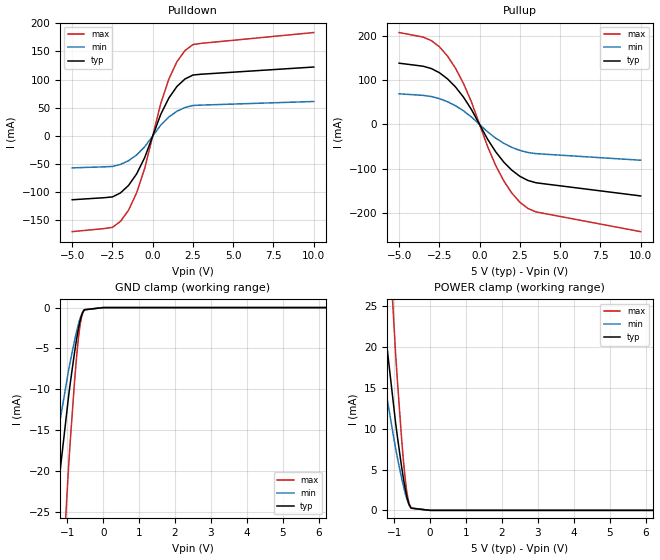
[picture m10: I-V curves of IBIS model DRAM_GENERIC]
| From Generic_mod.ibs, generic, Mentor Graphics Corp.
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[Model]   DRAM_GENERIC
Model_type   I/O
Polarity   Non-Inverting
Vinl  =   0.800V
Vinh  =   2.000V
Vmeas =   1.500V
Cref  =  50.000pF
Rref  =   1.000kOhm
Vref  =   0.000V
|   typ   min   max
C_comp   5.000pF   2.500pF   7.500pF
[Voltage Range]   5.000V   4.500V   5.500V
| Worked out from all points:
|   slope of the pulldown table from 0 to 0.75 V, typ, clamps not added: 14.2 ohm
|   slope of the pullup table from 0 to 0.75 V, typ, clamps not added: 15.8 ohm
|   GND clamp passes 1 mA (typ) near -0.61 V on its own axis
|   POWER clamp passes 1 mA (typ) near -0.61 V on its own axis
[Pulldown]
| Voltage   I(typ)   I(min)   I(max)
-5V       -113.2mA   -56.6mA    -169.8mA
-2.5V     -108.2mA   -54.08mA   -162.2mA
-2V       -101mA     -50.51mA   -151.5mA
-1.5V     -87.75mA   -43.88mA   -131.6mA
-1V       -67.27mA   -33.64mA   -100.9mA
-500mV    -38.46mA   -19.23mA   -57.69mA
500mV     38.46mA    19.23mA    57.69mA
1V        67.27mA    33.64mA    100.9mA
1.5V      87.75mA    43.88mA    131.6mA
2V        101mA      50.51mA    151.5mA
3V        109.6mA    54.78mA    164.3mA
10V       122.4mA    61.18mA    183.5mA
[Pullup]
| Voltage   I(typ)   I(min)   I(max)
-5V       137.8mA    68.9mA     206.7mA
-3V       125.8mA    62.89mA    188.7mA
-2V       102.8mA    51.38mA    154.1mA
-1.5V     84.46mA    42.23mA    126.7mA
-1V       61.41mA    30.7mA     92.11mA
-500mV    33.33mA    16.67mA    50mA
500mV     -33.33mA   -16.67mA   -50mA
1V        -61.41mA   -30.7mA    -92.11mA
1.5V      -84.46mA   -42.23mA   -126.7mA
2.5V      -116.5mA   -58.23mA   -174.7mA
3.5V      -130.9mA   -65.46mA   -196.4mA
10V       -160.6mA   -80.28mA   -240.8mA
[GND Clamp]
| Voltage   I(typ)   I(min)   I(max)
-5V       -167mA     -111.9mA   -331.4mA
-959.9mV  -10.66mA   -7.546mA   -19.1mA
-907.8mV  -8.916mA   -6.371mA   -15.68mA
-798.2mV  -5.465mA   -4.03mA    -9.021mA
-745.9mV  -3.978mA   -3.007mA   -6.241mA
-698.6mV  -2.774mA   -2.165mA   -4.08mA
-659mV    -1.905mA   -1.54mA    -2.61mA
-602.2mV  -952.4uA   -821.9uA   -1.159mA
-577.2mV  -658.6uA   -586.4uA   -761.9uA
-524.9mV  -269.3uA   -254uA     -287.6uA
0V        0A         0A         0A
10V       0A         0A         0A
[POWER Clamp]
| Voltage   I(typ)   I(min)   I(max)
-5V       167mA      111.9mA    331.4mA
-959.9mV  10.66mA    7.546mA    19.1mA
-907.8mV  8.916mA    6.371mA    15.68mA
-798.2mV  5.465mA    4.03mA     9.021mA
-745.9mV  3.978mA    3.007mA    6.241mA
-698.6mV  2.774mA    2.165mA    4.08mA
-659mV    1.905mA    1.54mA     2.61mA
-602.2mV  952.4uA    821.9uA    1.159mA
-577.2mV  658.6uA    586.4uA    761.9uA
-524.9mV  269.3uA    254uA      287.6uA
0V        0A         0A         0A
10V       0A         0A         0A
[Ramp]
|   typ   min   max
dV/dt_r   2.231V/2.700ns   1.522V/4.860ns   2.712V/1.980ns
dV/dt_f   2.275V/2.700ns   1.509V/4.860ns   2.761V/1.980ns
R_load =  50.000Ohm
|------------------- End of DRAM_GENERIC --------------------------------------
